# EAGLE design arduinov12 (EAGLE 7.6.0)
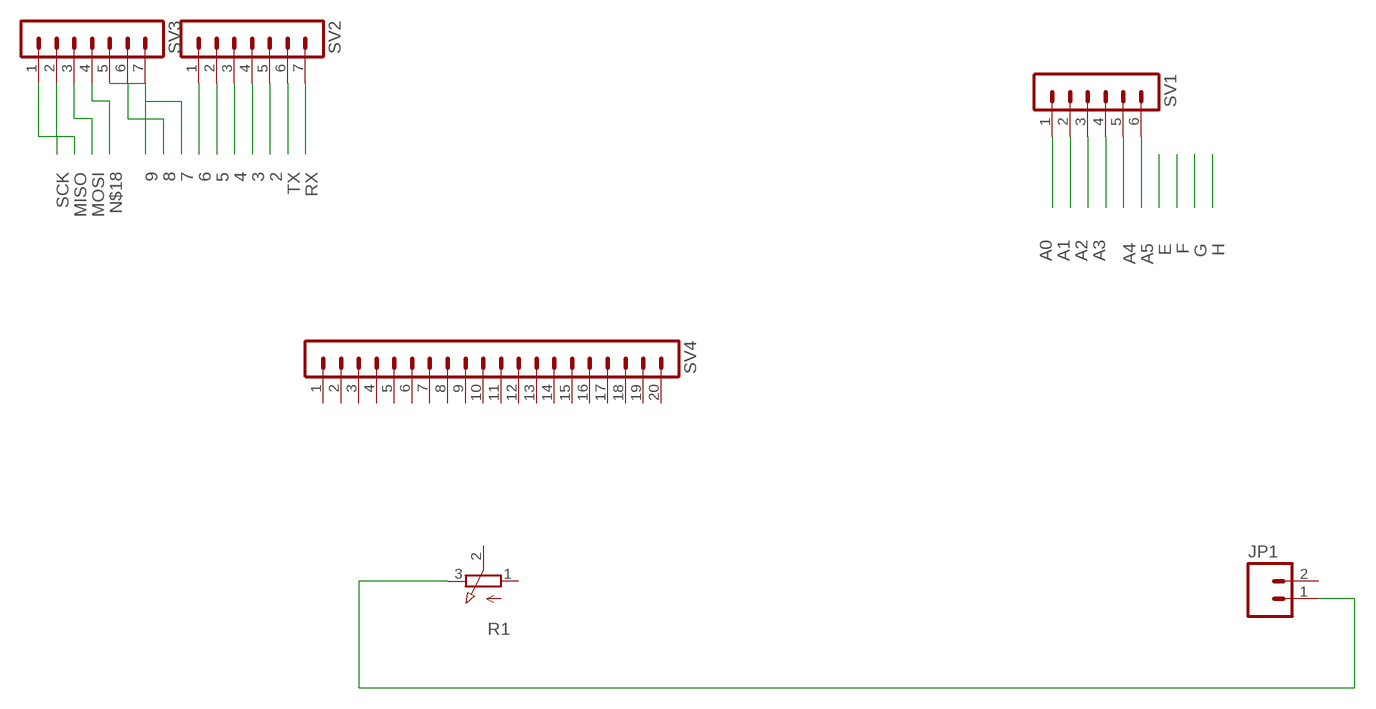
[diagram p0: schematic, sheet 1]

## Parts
JP1  M02LOCK_LONGPADS  [1X02_LOCK_LONGPADS]
R1  3RP/1610N  [3RP/1610N]
SV1  MA06-1  [MA06-1]
SV2  MA07-1  [MA07-1]
SV3  MA07-1  [MA07-1]
SV4  MA20-1  [MA20-1]

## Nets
2: SV2.5
3: SV2.4
4: SV2.3
5: SV2.2
6: SV2.1
7: SV3.7
8: SV3.6
9: SV3.5
A0: SV1.1
A1: SV1.2
A2: SV1.3
A3: SV1.4
A4: SV1.5
A5: SV1.6
MISO: SV3.2
MOSI: SV3.3
N$4: JP1.1 R1.3(E)
N$18: SV3.4
RX: SV2.7
SCK: SV3.1
TX: SV2.6
Unconnected: JP1.2 R1.1(A) R1.2(S) SV4.1 SV4.2 SV4.3 SV4.4 SV4.5 SV4.6 SV4.7 SV4.8 SV4.9 SV4.10 SV4.11 SV4.12 SV4.13 SV4.14 SV4.15 SV4.16 SV4.17 SV4.18 SV4.19 SV4.20

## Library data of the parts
JP1 = SparkFun:M02: Header 2
R1 = pot:3RP/1610N: 16mm Potentiometer one level Source: http://www.alphapotentiometers.net/html/16mm_pot_2.html
SV1 = con-lstb:MA06-1: PIN HEADER; OC_FARNELL: unknown; OC_NEWARK: unknown
SV2 SV3 = con-lstb:MA07-1: PIN HEADER; OC_FARNELL: unknown; OC_NEWARK: unknown
SV4 = con-lstb:MA20-1: PIN HEADER; OC_FARNELL: unknown; OC_NEWARK: unknown

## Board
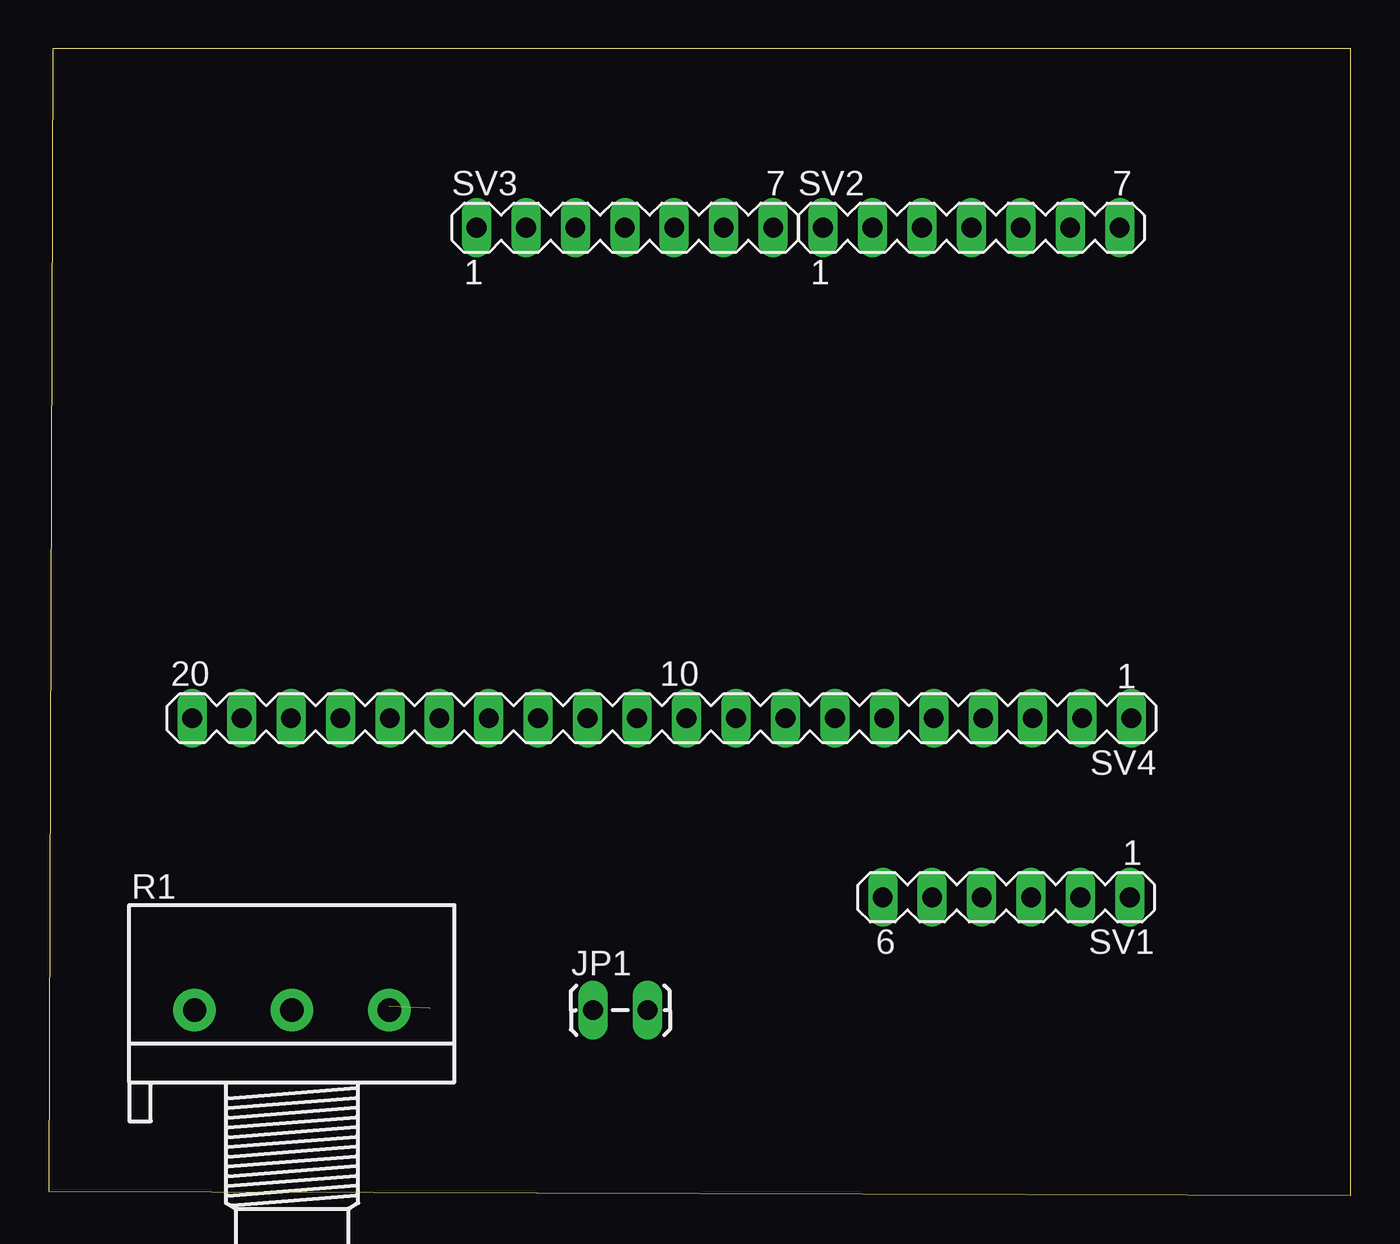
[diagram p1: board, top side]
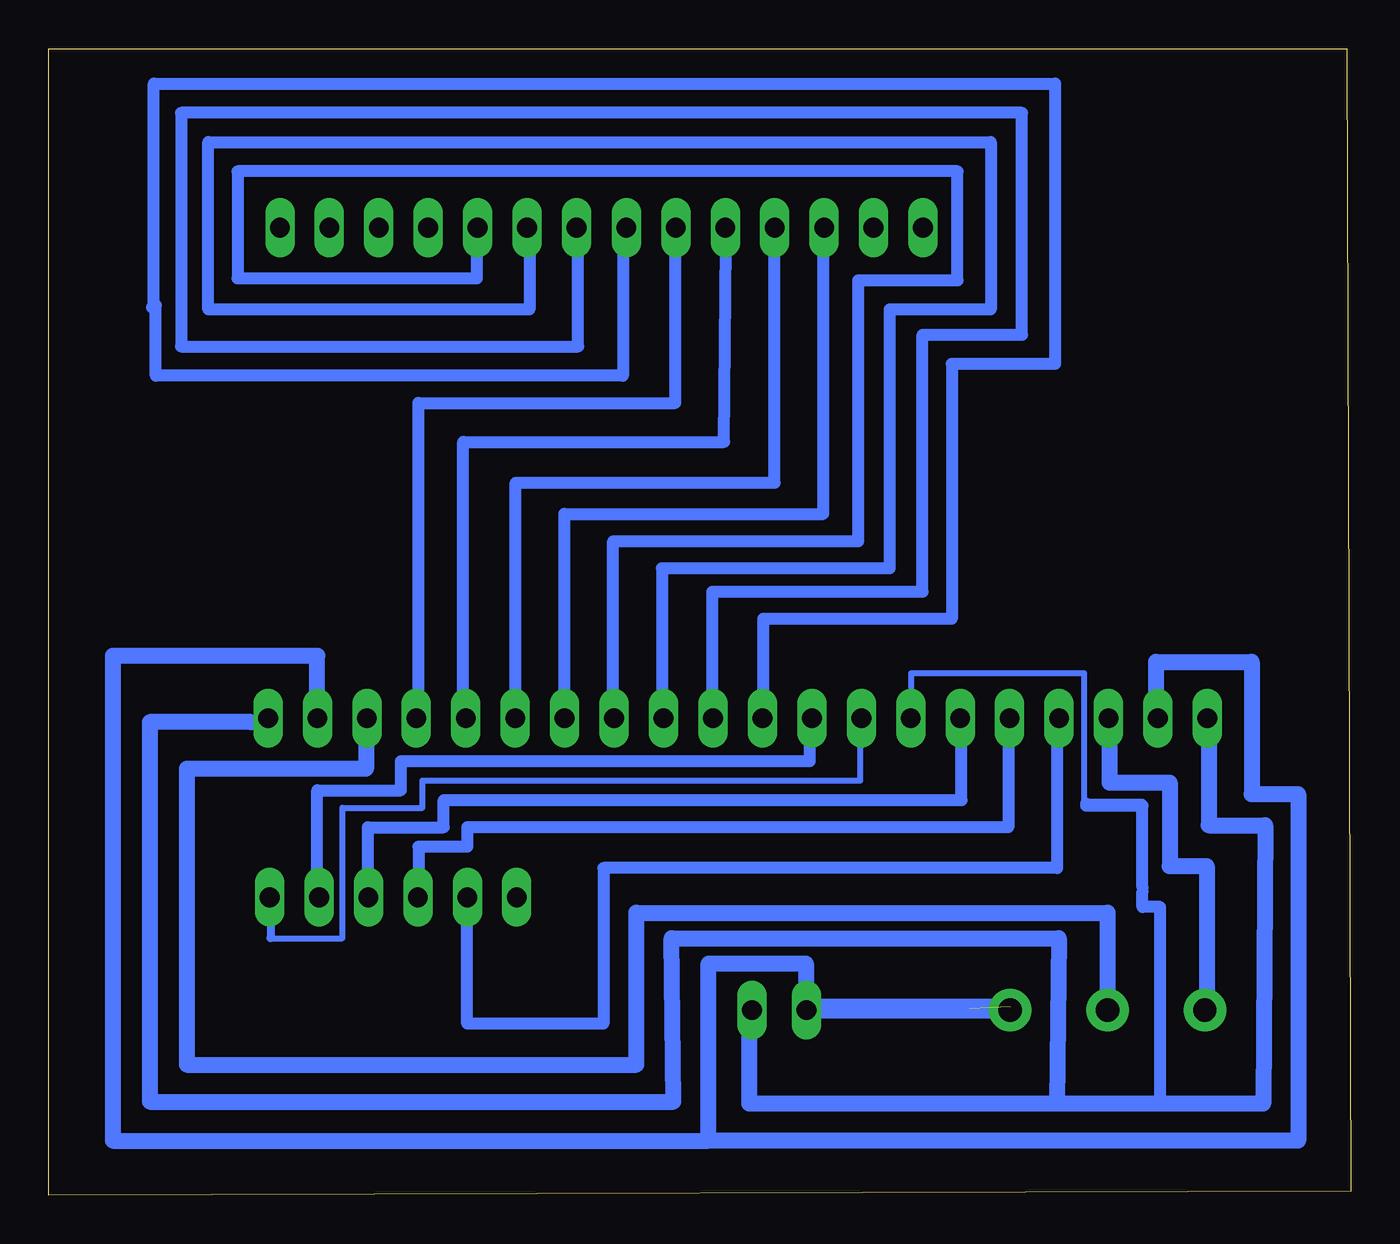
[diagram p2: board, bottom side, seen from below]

Size 66.9 x 58.9 mm. Coordinates in mm from the lower left corner, seen from the top.
Outline: 0,0.2 66.9,0 66.9,58.9 0.2,58.9 0,0.2
Copper layers (1*16): Top 0.035mm / dielectric 1.5mm / Bottom 0.035mm
Design rules "default": minimum track width 10mil, minimum drill 24mil, track to track 8mil, track to pad 8mil, pad to pad 8mil, via to via 8mil, smd to smd 8mil, copper to edge 40mil, drill to drill 8mil, minimum pad ring 10mil, minimum via ring 8mil, stop-mask expansion 4mil, vias tented up to drill 0mil, thermal gap 10mil

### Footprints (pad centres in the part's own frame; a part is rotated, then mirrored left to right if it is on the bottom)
1X02_LOCK_LONGPADS = drill 1.016 long: 1 -0.127,0; 2 2.667,0
3RP/1610N = drill 1.2 pad 2.184: 1 -5,0; 2 0,0; 3 5,0
MA06-1 = drill 1.016 long: 1 -6.35,0; 2 -3.81,0; 3 -1.27,0; 4 1.27,0; 5 3.81,0; 6 6.35,0
MA07-1 = drill 1.016 long: 1 -7.62,0; 2 -5.08,0; 3 -2.54,0; 4 0,0; 5 2.54,0; 6 5.08,0; 7 7.62,0
MA20-1 = drill 1.016 long: 1 -24.13,0; 2 -21.59,0; 3 -19.05,0; 4 -16.51,0; 5 -13.97,0; 6 -11.43,0; 7 -8.89,0; 8 -6.35,0; 9 -3.81,0; 10 -1.27,0; 11 1.27,0; 12 3.81,0; 13 6.35,0; 14 8.89,0; 15 11.43,0; 16 13.97,0; 17 16.51,0; 18 19.05,0; 19 21.59,0; 20 24.13,0

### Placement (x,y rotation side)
JP1  28.1,9.5 0 top
R1  12.5,9.5 0 top
SV1  49.2,15.3 180 top
SV2  47.4,49.7 0 top
SV3  29.6,49.7 0 top
SV4  31.5,24.5 180 top

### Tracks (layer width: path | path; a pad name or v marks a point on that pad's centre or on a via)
N$4
  Bottom 0.813: JP1.1 R1.3
N$8  (1 unrouted)
  Bottom 0.813: 17.5,9.7 19.8,9.6 | 27.8,9.7 17.5,9.7 | 17.5,9.7 19.6,9.6
N$9
  Bottom 0.305: 55.5,13.2 51.8,13.2 51.8,19.9 47.7,19.9 47.7,21.3 25.2,21.3 25.2,23.8
  Bottom 0.406: 55.5,14.3 55.5,13.2
  Bottom 0.813: 55.6,14.3 55.5,14.3
N$10
  Bottom 0.813: 48,25.4 48.1,25.4
N$11
  Bottom 0.813: 43,25.6 42.9,25.6
N$12
  Bottom 0.813: 12.5,23.5 12.4,23.6 12.4,21.2 9.3,21.2 9.3,16.9 7.4,16.9 7.4,10.3
N$13
  Bottom 0.813: 56.5,24.3 61.7,24.3 61.7,4.8 34.8,4.8 34.9,13.2 15,13.2 15.1,4.7 | 7.3,23.5 7.3,19 4.4,19 4.5,4.7 15.1,4.7 | 15.1,4.7 30.9,4.7 30.9,9.5
N$14
  Bottom 0.813: 53,25.4 53.1,25.4 53.1,27.7 63.6,27.7 63.6,2.8 33,2.8 | 10,25.5 10,27.4 5.1,27.4 5.1,20.6 2.7,20.6 2.7,2.8 33,2.8 | 33,2.8 33,11.9 28,11.9 28,9.5
N$15
  Bottom 0.813: 50.6,23.6 50.6,21.9 59.8,21.9 59.8,6.7 36.7,6.7 36.7,14.5 12.5,14.5 12.5,10.3
N$16
  Bottom 0.61: 48,25.4 47.9,25.5 47.9,40.7 34.7,40.7 34.7,48.9
N$17
  Bottom 0.61: 45.6,25.5 45.6,38.7 32.2,38.7 32.1,48.8
N$18
  Bottom 0.61: 43,25.4 42.9,25.7 42.9,36.6 29.6,36.6 SV3.4
N$19
  Bottom 0.61: 40.4,25.4 40.4,35 27.1,35 27.1,48.9
N$20
  Bottom 0.61: 37.9,25.4 37.9,33.6 25.3,33.6 25.3,47 20.2,47 20.2,52.6 57.2,52.6 57.2,47.1 44.9,47.1 44.9,48.8
N$21
  Bottom 0.61: 42.3,48.7 42.2,48.7 42.2,45.5 58.7,45.5 58.7,54.1 18.5,54.1 18.5,45.5 23.7,45.5 23.7,32.2 35.4,32.2 35.4,25.3
N$22
  Bottom 0.61: 32.8,25.5 32.8,31 22,31 22,44.2 16.9,44.2 16.9,55.6 60.1,55.6 60.1,43.6 39.7,43.6 39.7,48.9
N$23
  Bottom 0.61: 37.3,48.7 37.4,48.5 37.4,42.1 61.4,42.1 61.4,45.7
N$24
  Bottom 0.61: 61.6,45.6 61.5,45.6 61.5,57.1 15.2,57.1 15.2,42.7 20.5,42.7 20.5,29.6 30.2,29.6 30.2,25.3
N$25
  Bottom 0.61: 53.1,16.2 53.1,20.8 48.8,20.8 48.8,22.3 27.8,22.3 27.8,23.6
N$26
  Bottom 0.61: 55.6,14.1 55.7,14.3
N$27
  Bottom 0.61: 9.6,4.6 9.8,4.6 9.8,14.8 10.7,14.8 10.7,15.6
N$28
  Bottom 0.305: 10.7,20 10.7,20.2 13.7,20.2 13.7,26.8 22.6,26.8 22.6,25.1
  Bottom 0.61: 10.7,15.8 10.7,20 13.6,20 13.6,20.1
N$29
  Bottom 0.61: 50.5,16.3 50.5,18.9 46.6,18.9 46.6,20.3 20,20.3 20,23.7
N$30
  Bottom 0.61: 17.6,23.6 17.6,18.9 45.4,18.9 45.4,17.9 47.9,17.9 47.9,16.1
N$31
  Bottom 0.61: 15.1,23.7 15.1,16.8 38.4,16.8 38.4,8.8 45.4,8.8 45.4,14.4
